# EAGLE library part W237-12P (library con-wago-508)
WAGO SREW CLAMP
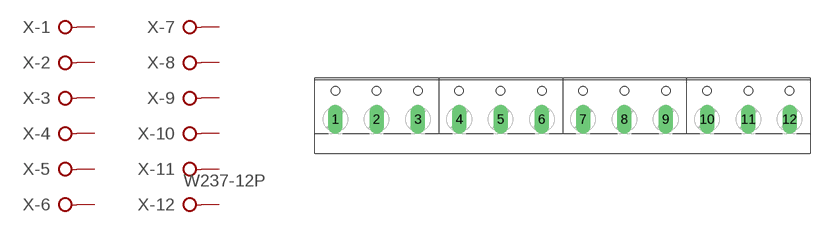
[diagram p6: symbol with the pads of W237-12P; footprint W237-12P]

Designator prefix X; gates -1=KL -2=KL -3=KL -4=KL -5=KL -6=KL -7=KL -8=KL -9=KL -10=KL -11=KL -12=KL+V

## W237-12P (OC_FARNELL: unknown; OC_NEWARK: unknown)  [W237-12P]
1  -1:KL  pas
2  -2:KL  pas
3  -3:KL  pas
4  -4:KL  pas
5  -5:KL  pas
6  -6:KL  pas
7  -7:KL  pas
8  -8:KL  pas
9  -9:KL  pas
10  -10:KL  pas
11  -11:KL  pas
12  -12:KL  pas

## Footprint W237-12P (pad centres in mm)
WAGO SREW CLAMP
drill 1.194 long: 1 -27.94,-0.635; 2 -22.86,-0.635; 3 -17.78,-0.635; 4 -12.7,-0.635; 5 -7.62,-0.635; 6 -2.54,-0.635; 7 2.54,-0.635; 8 7.62,-0.635; 9 12.7,-0.635; 10 17.78,-0.635; 11 22.86,-0.635; 12 27.94,-0.635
